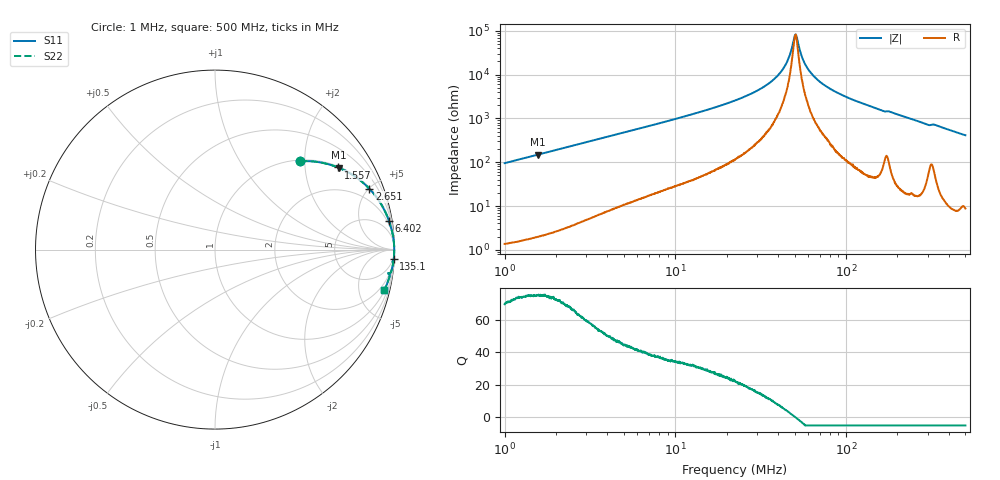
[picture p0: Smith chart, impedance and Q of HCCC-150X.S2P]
!s-Parameter Generated by FASTRON Sdn. Bhd.
!FASTRON P/N : HCCC-150X
!Keysight Technologies,E4991B,MY54100416,A.01.15
!Date: Mon Apr 06 13:29:25 2026
!Version  : Rev00 Mon Apr 06 13:29:25 2026
!Data & Calibration Information:
!PortZ  Port1:50+j0  Port2:50+j0
!When reading, reference impedance value at option line is always used.
! Remarks : This data is being provided solely for informational purposes.
!Freq	S11	S21	S12	S22
# Hz S dB R 50
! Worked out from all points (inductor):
!   1601 points, 1 MHz to 500 MHz, reference 50 ohm
!   read as one part in series: L = 15.1 uH near 1.032 MHz
!   highest Q = 75.3 at 1.575 MHz (marker M1), where L = 15.1 uH
!   self-resonance near 50.55 MHz
!   S11 on the Smith chart (normalised r, x): 1 MHz: 1.03, +1.90; 1.557 MHz: 1.04, +2.96; 2.651 MHz: 1.08, +5.05; 6.402 MHz: 1, +12; 135.1 MHz: 2, -39; 500 MHz: 1.18, -8.26
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1000000  -3.29 46.0  -2.86 -43.2  -2.86 -43.2  -3.29 46.0
1557047  -1.68 33.8  -5.10 -55.5  -5.10 -55.5  -1.68 33.8
1575296  -1.65 33.5  -5.17 -55.8  -5.17 -55.8  -1.65 33.5
2650946  -0.68 21.5  -8.72 -67.6  -8.72 -67.6  -0.68 21.5
2820919  -0.61 20.3  -9.19 -68.8  -9.19 -68.8  -0.61 20.3
6402024  -0.15 9.2  -15.89 -79.3  -15.89 -79.3  -0.15 9.2
7957584  -0.10 7.4  -17.78 -81.0  -17.78 -81.0  -0.10 7.4
2.236068e7  -0.02 2.2  -28.22 -85.2  -28.22 -85.2  -0.02 2.2
3.159477e7  -0.01 1.2  -33.58 -84.9  -33.58 -84.9  -0.01 1.2
3.942448e7  -0.01 0.6  -39.26 -82.3  -39.26 -82.3  -0.01 0.6
4.516541e7  -0.01 0.3  -45.93 -75.7  -45.93 -75.7  -0.01 0.3
4.695421e7  -0.01 0.2  -49.22 -68.4  -49.22 -68.4  -0.01 0.2
4.938598e7  -0.01 0.1  -55.88 -39.1  -55.88 -39.1  -0.01 0.1
5.055043e7  -0.01 0.0  -58.32 -3.4  -58.32 -3.4  -0.01 0.0
5.174233e7  -0.01 -0.1  -56.29 39.6  -56.29 39.6  -0.01 -0.1
5.442207e7  -0.01 -0.2  -49.52 69.0  -49.52 69.0  -0.01 -0.2
5.679767e7  -0.01 -0.3  -45.71 76.6  -45.71 76.6  -0.01 -0.3
6.307767e7  -0.01 -0.6  -40.25 82.7  -40.25 82.7  -0.01 -0.6
8.343135e7  -0.01 -1.3  -32.91 85.7  -32.91 85.7  -0.01 -1.3
1.350515e8  -0.02 -2.9  -25.90 85.7  -25.90 85.7  -0.02 -2.9
1.77937e8  -0.06 -3.9  -23.28 82.1  -23.28 82.1  -0.06 -3.9
5e8  -0.29 -13.5  -12.61 75.2  -12.61 75.2  -0.29 -13.5
